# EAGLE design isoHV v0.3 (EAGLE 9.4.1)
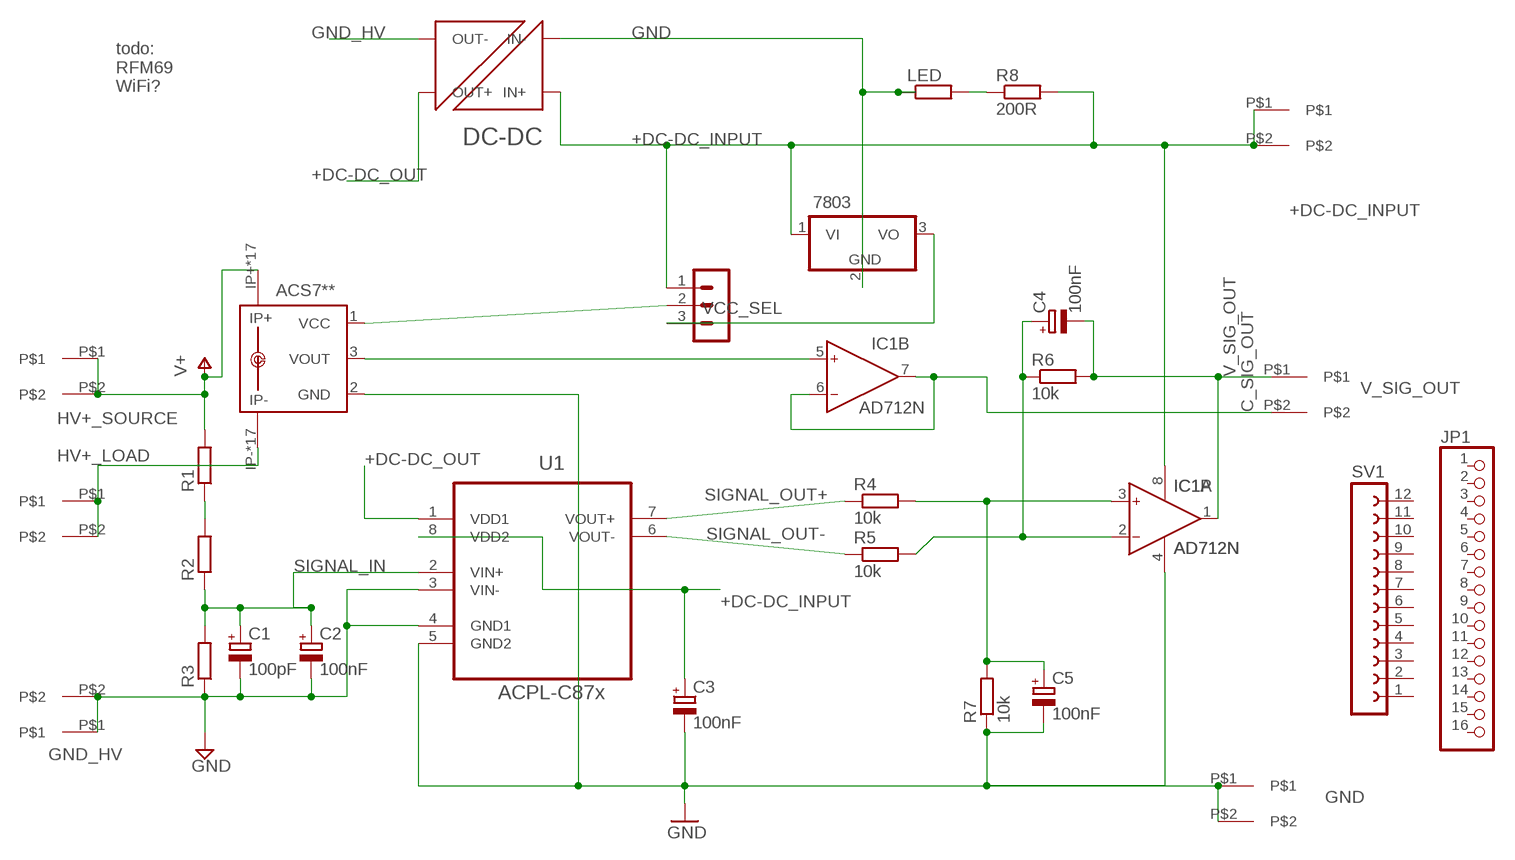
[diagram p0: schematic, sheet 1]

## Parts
7803  7805TV  [TO220V]
ACS7**  ACS758KCB-150B-PFF-T  [CB-PFF]
C1  100pF  CPOL-EUB45181A  [B45181A]
C2  100nF  CPOL-EUB45181A  [B45181A]
C3  100nF  CPOL-EUB45181A  [B45181A]
C4  100nF  CPOL-EUB45181A  [B45181A]
C5  100nF  CPOL-EUB45181A  [B45181A]
IC1  AD712N  [DIL08]
JP1  HEADER-1X16  [1X16_OVAL]
LED  R-EU_0204/2V  [0204V]
R1  R-EU_0411/15  [0411/15]
R2  R-EU_0411/15  [0411/15]
R3  R-EU_0411/15  [0411/15]
R4  10k  R-EU_0204/7  [0204/7]
R5  10k  R-EU_0204/7  [0204/7]
R6  10k  R-EU_0204/7  [0204/7]
R7  10k  R-EU_0204/7  [0204/7]
R8  200R  R-EU_0204/2V  [0204V]
SV1  FE12-1  [FE12]
U1  ACPL-C87x  ACPL-C79B-000E  [SOIC127P1150X330-8N]
U$1  7.62MM_TERMINAL_BLOCK  [7.62MM]
U$2  7.62MM_TERMINAL_BLOCK  [7.62MM]
U$3  7.62MM_TERMINAL_BLOCK  [7.62MM]
U$4  7.62MM_TERMINAL_BLOCK  [7.62MM]
U$5  7.62MM_TERMINAL_BLOCK  [7.62MM]
U$6  7.62MM_TERMINAL_BLOCK  [7.62MM]
U$7  NXF1  [NXF1]
VCC_SEL  MA03-1  [MA03-1]

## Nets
+DC-DC_INPUT: 7803.1(VI) C3.+ IC1.8(P:V+) R8.2 U1.8(VDD2) U$3.P$1 U$3.P$2 U$7.P$3(IN+) VCC_SEL.1
+DC-DC_OUT: U1.1(VDD1) U$7.P$8(OUT+)
C_SIG_OUT: IC1.6(B:IN-) IC1.7(B:OUT) U$5.P$2
GND: 7803.2(GND) ACS7**.2(GND) C3.- C5.- IC1.4(P:V-) LED.1 R7.1 U1.5(GND2) U$4.P$1 U$4.P$2 U$7.P$1(IN-)
GND_HV: C1.- C2.- R3.1 U1.3(VIN-) U1.4(GND1) U$2.P$1 U$2.P$2 U$7.P$7(OUT-) ; supply symbol labelled GND
HV+_LOAD: ACS7**.IP- ACS7**.IP-@2(IP-) ACS7**.IP-@3(IP-) ACS7**.IP-@4(IP-) ACS7**.IP-@5(IP-) ACS7**.IP-@6(IP-) ACS7**.IP-@7(IP-) ACS7**.IP-@8(IP-) ACS7**.IP-@9(IP-) ACS7**.IP-@10(IP-) ACS7**.IP-@11(IP-) ACS7**.IP-@12(IP-) ACS7**.IP-@13(IP-) ACS7**.IP-@14(IP-) ACS7**.IP-@15(IP-) ACS7**.IP-@16(IP-) ACS7**.IP-@17(IP-) U$6.P$1 U$6.P$2
HV+_SOURCE: ACS7**.IP+ ACS7**.IP+@2(IP+) ACS7**.IP+@3(IP+) ACS7**.IP+@4(IP+) ACS7**.IP+@5(IP+) ACS7**.IP+@6(IP+) ACS7**.IP+@7(IP+) ACS7**.IP+@8(IP+) ACS7**.IP+@9(IP+) ACS7**.IP+@10(IP+) ACS7**.IP+@11(IP+) ACS7**.IP+@12(IP+) ACS7**.IP+@13(IP+) ACS7**.IP+@14(IP+) ACS7**.IP+@15(IP+) ACS7**.IP+@16(IP+) ACS7**.IP+@17(IP+) R1.2 U$1.P$1 U$1.P$2 ; supply symbol labelled V+
N$1: C5.+ IC1.3(A:IN+) R4.2 R7.2
N$2: R1.1 R2.2
N$3: ACS7**.1(VCC) VCC_SEL.2
N$4: LED.2 R8.1
N$5: C4.+ IC1.2(A:IN-) R5.2 R6.1
N$6: ACS7**.3(VOUT) IC1.5(B:IN+)
N$7: 7803.3(VO) VCC_SEL.3
SIGNAL_IN: C1.+ C2.+ R2.1 R3.2 U1.2(VIN+)
SIGNAL_OUT+: R4.1 U1.7(VOUT+)
SIGNAL_OUT-: R5.1 U1.6(VOUT-)
V_SIG_OUT: C4.- IC1.1(A:OUT) R6.2 U$5.P$1
Unconnected: JP1.1 JP1.2 JP1.3 JP1.4 JP1.5 JP1.6 JP1.7 JP1.8 JP1.9 JP1.10 JP1.11 JP1.12 JP1.13 JP1.14 JP1.15 JP1.16 SV1.1 SV1.2 SV1.3 SV1.4 SV1.5 SV1.6 SV1.7 SV1.8 SV1.9 SV1.10 SV1.11 SV1.12

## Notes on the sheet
- todo:
  RFM69
  WiFi?

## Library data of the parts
7803 = linear:78*: Positive VOLTAGE REGULATOR Source: http://cache.national.com/ds/LM/LM78L05.pdf http://www.fairchildsemi.com/ds/LM/LM7805.pdf
ACS7** = allegro:ACS758*: Thermally Enhanced, Fully Integrated, Hall Effect-Based Linear Current Sensor with 100 micro Ohm Current Conductor display layer 49 Reference in BRD and place VIAs on circles Source: http://www.allegromicro.com/en/Products/Part_Numbers/0758/0758.pdf; MPN: ACS7**; OC_FARNELL: 1718995; OC_NEWARK: 04R7129
C1-C5 = rcl:CPOL-EU: POLARIZED CAPACITOR, European symbol; SPICEPREFIX: C
IC1 = analog-devices:AD712: Dual Precision, Low Cost, High Speed BiFET Op Amp Source: http://www.analog.com/static/imported-files/data_sheets/AD712.pdf; MF: ALTERA CORPORATION; MPN: AD712JNZ; OC_FARNELL: 9604898; OC_NEWARK: 59K4554
JP1 = microbuilder:HEADER-1X16: PIN HEADER
LED R1-R8 = rcl:R-EU_: RESISTOR, European symbol; SPICEPREFIX: R
SV1 = con-lsta-RFM69Pi:FE12-1: FEMALE HEADER; OC_FARNELL: unknown; OC_NEWARK: unknown
U1 = Avago_By_element14_Batch_1:ACPL-C79B-000E: Precision Miniature Isolation Amplifiers; DESCRIPTION: Precision Miniature Isolation Amplifiers; MPN: ACPL-C79B-000E; OC_FARNELL: 1854253; OC_NEWARK: 74R5803; PACKAGE: SOIC-8; SUPPLIER: AVAGO TECHNOLOGIES
U$1-U$6 = 7.62mm terminal block:7.62MM_TERMINAL_BLOCK
U$7 = NXF1:NXF1
VCC_SEL = con-lstb:MA03-1: PIN HEADER; OC_FARNELL: unknown; OC_NEWARK: unknown

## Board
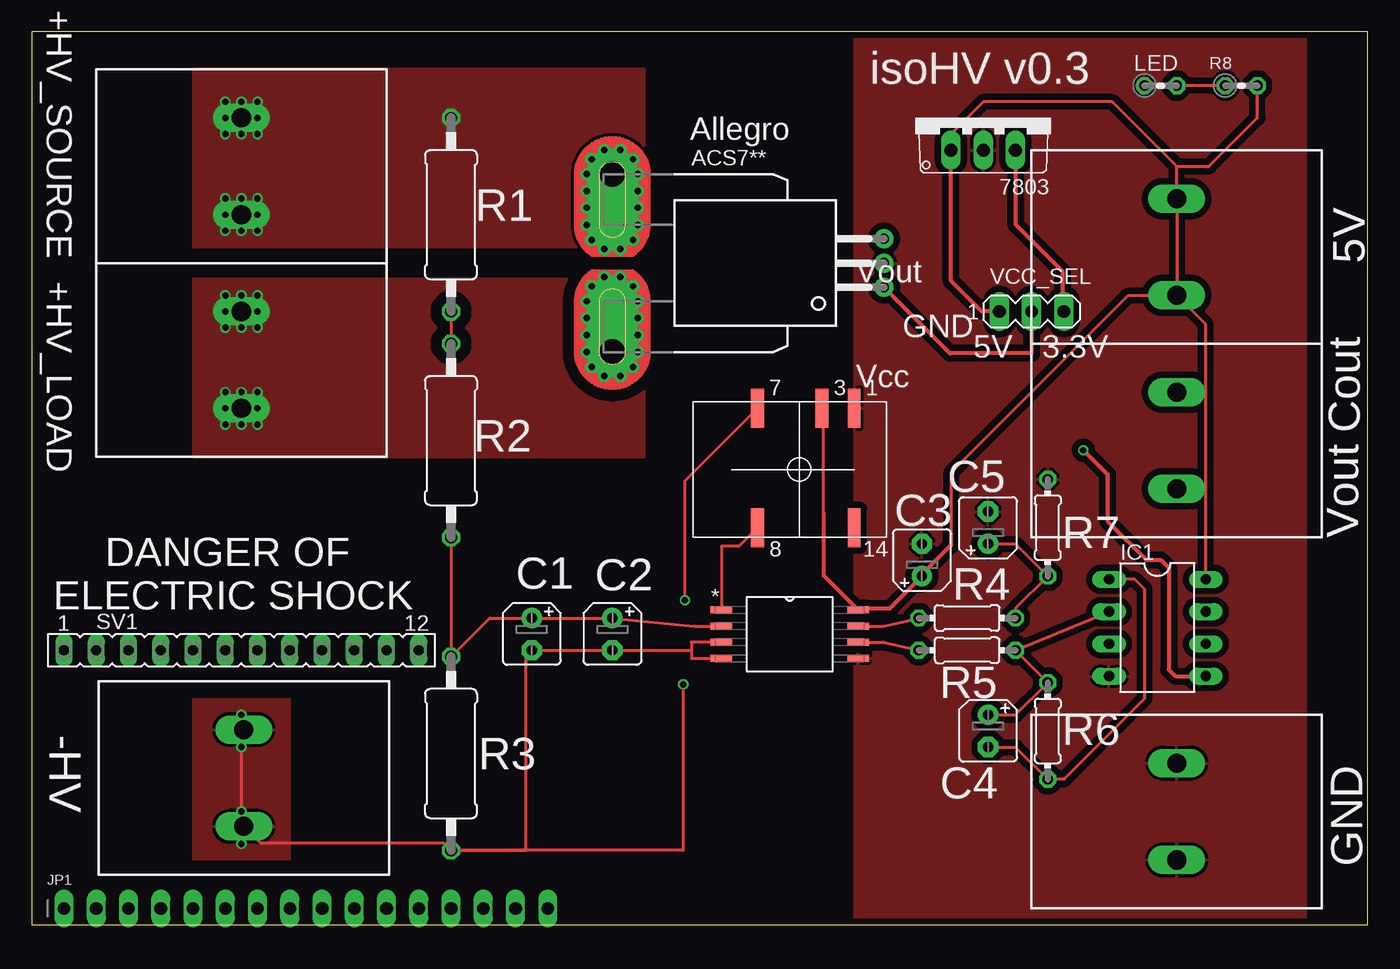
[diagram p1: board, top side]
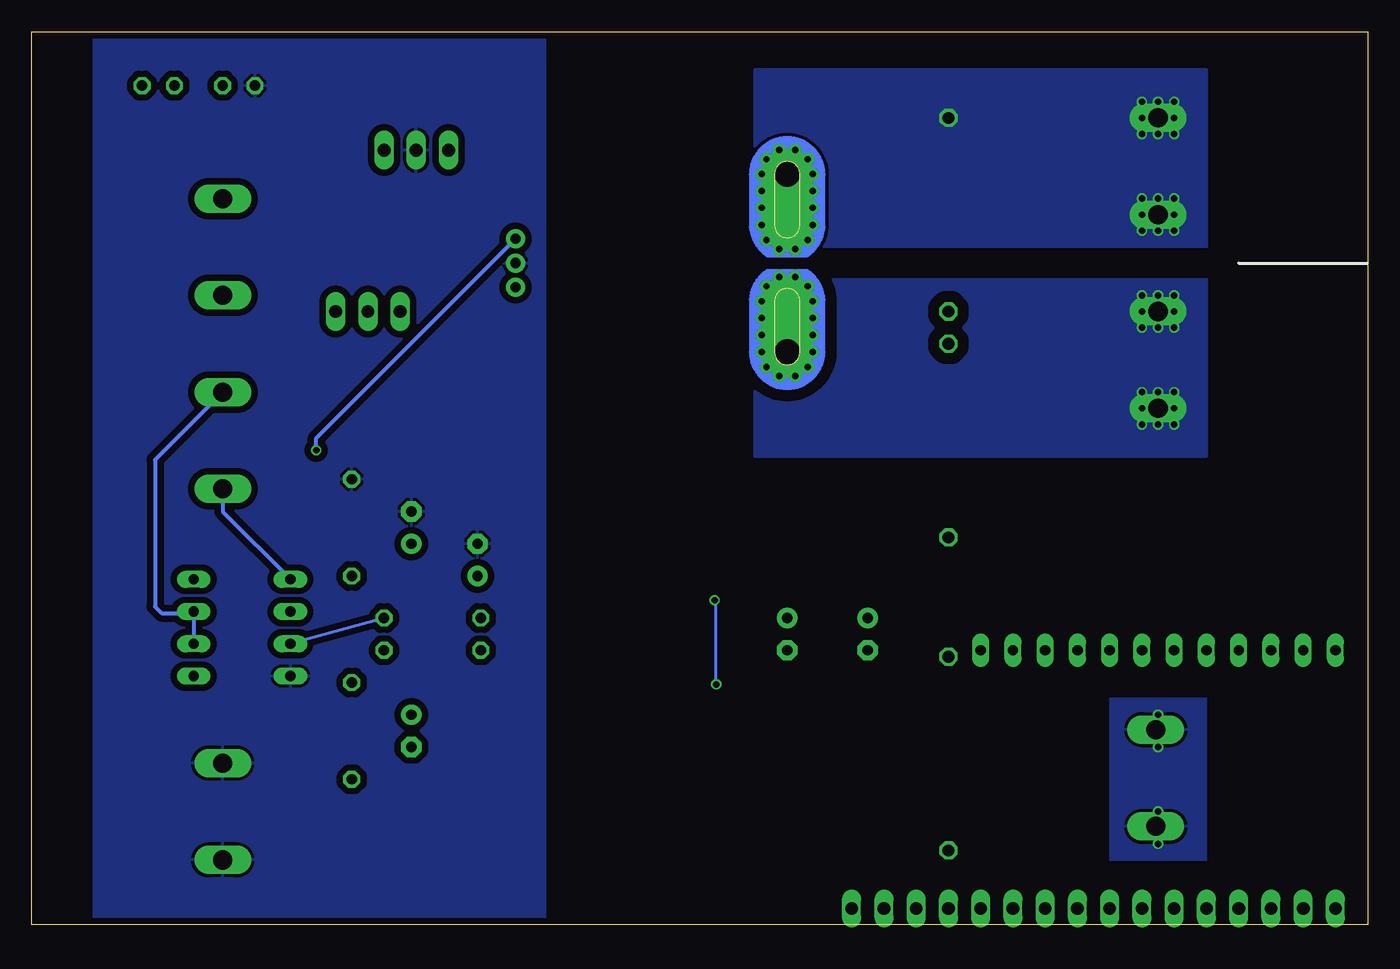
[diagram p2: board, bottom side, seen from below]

Size 105.21 x 70.28 mm. Coordinates in mm from the lower left corner, seen from the top.
Outline: 0,70.28 0,0 105.21,0 105.21,70.28 0,70.28
Copper layers (1*16): Top 0.07111875mm / dielectric 1.45776875mm / Bottom 0.07111875mm
Design rules "jlcpcb *": minimum track width 6mil, minimum drill 12mil, track to track 10mil, track to pad 10mil, pad to pad 10mil, via to via 10mil, smd to smd 0mil, copper to edge 10mil, drill to drill 10mil, minimum pad ring 10mil, minimum via ring 6mil, stop-mask expansion 2mil, vias tented up to drill 25mil, thermal gap 10mil

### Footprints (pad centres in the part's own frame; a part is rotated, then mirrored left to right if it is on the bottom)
TO220V = drill 1.016 long: 1 -2.54,-2.54; 2 0,-2.54; 3 2.54,-2.54
CB-PFF = drill 0.8 pad 1.5: 1 -1.91,-21.4; 2 0,-21.4; 3 1.91,-21.4 | drill 2 pad 4 offset: IP+ 7,0; IP- -7,0 | drill 0.5 pad 0.9: IP+@2 8.89,0.635; IP+@3 8.89,-0.635; IP+@4 8.175,-1.625; IP+@5 7,-2; IP+@6 5.675,-2; IP+@7 4.35,-2; IP+@8 3,-2; IP+@9 1.825,-1.625; IP+@10 1.1,-0.625; IP+@11 1.1,0.625; IP+@12 1.825,1.625; IP+@13 3,2; IP+@14 4.35,2; IP+@15 5.675,2; IP+@16 7,2; IP+@17 8.175,1.625; IP-@2 -8.89,0.635; IP-@3 -8.89,-0.635; IP-@4 -8.175,-1.625; IP-@5 -7,-2; IP-@6 -5.675,-2; IP-@7 -4.325,-2; IP-@8 -3,-2; IP-@9 -1.825,-1.625; IP-@10 -1.1,-0.625; IP-@11 -1.1,0.625; IP-@12 -1.825,1.625; IP-@13 -3,2; IP-@14 -4.325,2; IP-@15 -5.675,2; IP-@16 -7,2; IP-@17 -8.175,1.625
B45181A = drill 0.813 pad 1.6: + -1.27,0 | drill 0.813 pad 1.6 octagon: - 1.27,0
DIL08 = drill 0.813 long: 1 -3.81,-3.81; 2 -1.27,-3.81; 3 1.27,-3.81; 4 3.81,-3.81; 5 3.81,3.81; 6 1.27,3.81; 7 -1.27,3.81; 8 -3.81,3.81
1X16_OVAL = drill 1 long: 1 -19.05,0; 2 -16.51,0; 3 -13.97,0; 4 -11.43,0; 5 -8.89,0; 6 -6.35,0; 7 -3.81,0; 8 -1.27,0; 9 1.27,0; 10 3.81,0; 11 6.35,0; 12 8.89,0; 13 11.43,0; 14 13.97,0; 15 16.51,0; 16 19.05,0
0204V = drill 0.813 octagon: 1 -1.27,0; 2 1.27,0
0411/15 = drill 0.914 octagon: 1 -7.62,0; 2 7.62,0
0204/7 = drill 0.813 octagon: 1 -3.81,0; 2 3.81,0
FE12 = drill 0.813 long: 1 -13.97,0; 2 -11.43,0; 3 -8.89,0; 4 -6.35,0; 5 -3.81,0; 6 -1.27,0; 7 1.27,0; 8 3.81,0; 9 6.35,0; 10 8.89,0; 11 11.43,0; 12 13.97,0
SOIC127P1150X330-8N = smd 1.702 x 0.559: 1 -5.385,1.905; 2 -5.385,0.635; 3 -5.385,-0.635; 4 -5.385,-1.905; 5 5.385,-1.905; 6 5.385,-0.635; 7 5.385,0.635; 8 5.385,1.905
7.62MM = drill 1.5 long: P$1 0,-3.81; P$2 0,3.81
NXF1 = smd 0.991 x 3.048: P$1 0,0; P$3 2.54,0; P$7 7.62,0; P$8 7.62,9.398; P$14 0,9.398
MA03-1 = drill 1.016 long: 1 -2.54,0; 2 0,0; 3 2.54,0

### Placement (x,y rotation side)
7803  74.93,63.5 0 top
ACS7**  45.72,52.07 90 top
C1  39.37,22.86 270 top
C2  45.72,22.86 270 top
C3  70.1,28.7 90 top
C4  75.31,15.24 270 top
C5  75.31,31.24 90 top
IC1  88.65,23.37 270 top
JP1  21.59,1.27 0 top
LED  88.9,66.04 0 top
R1  33.02,55.88 90 top
R2  33.02,38.1 90 top
R3  33.02,13.46 90 top
R4  73.66,24.13 0 top
R5  73.66,21.59 0 top
R6  80.01,15.24 270 top
R7  80.01,31.24 270 top
R8  95.25,66.04 0 top
SV1  16.51,21.59 0 top
U1  59.69,22.86 0 top
U$1  16.51,59.69 180 top
U$2  16.7,11.54 0 top
U$3  90.17,53.34 0 top
U$4  90.17,8.89 180 top
U$5  90.17,38.1 0 top
U$6  16.51,44.45 0 top
U$7  64.77,40.64 180 top
VCC_SEL  78.74,48.26 0 top

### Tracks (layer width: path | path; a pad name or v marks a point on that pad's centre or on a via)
+DC-DC_INPUT
  Top 0.254: 65.08,24.88 U1.8 | IC1.8 92.46,47.24 U$3.P$1 | U$3.P$1 U$3.P$2 90.17,59.69 | 72.39,30.73 72.39,35.56 86.36,49.53 U$3.P$1 | 90.17,59.69 85.09,64.77 74.93,64.77 72.39,62.23 7803.1 | 62.36,30.48 62.36,40.51 U$7.P$3 | 90.17,59.69 92.71,59.69 96.52,63.5 R8.2
  Top 0.305: 7803.1 72.39,50.67 74.8,48.26 VCC_SEL.1 | 72.39,30.73 72.39,29.84 70.1,27.56 C3.+ 67.55,24.88 65.08,24.88 | U1.8 62.36,27.48 62.36,30.48 62.36,32.37
+DC-DC_OUT
  Top 0.254: U1.1 54.3,29.77 55.68,29.77 U$7.P$8
C_SIG_OUT
  Bottom 0.305: U$5.P$2 95.5,36.58 95.5,25.02 95,24.51 92.58,24.51 IC1.7 IC1.6
GND
  pour Bottom (isolate 0.508): 100.33,71.12 100.33,0 64.77,0 64.77,71.12
  pour Top (isolate 0.508): 64.77,71.12 64.77,0 100.33,0 100.33,71.12
GND_HV  (via drill 0.5)
  Top 0.254: U1.3 51.94,22.23 51.94,21.59 | 51.94,21.59 51.94,20.95 U1.4 | U$2.P$2 16.7,14.16 v16.51,13.97 v16.51,8.89 16.7,8.7 U$2.P$1 18.04,6.39 32.47,6.39 R3.1 | R3.1 38.9,5.84 38.9,21.12 C1.- C2.- 51.94,21.59 | R3.1 51.31,5.84 v51.31,18.9 | v51.44,25.53 51.44,34.92 U$7.P$7
  Bottom 0.254: v51.31,18.9 51.31,25.4 v51.44,25.53
  other vias: 16.51,16.51 16.51,6.35
  pour Top: 12.7,17.78 20.32,17.78 20.32,5.08 12.7,5.08
  pour Bottom: 12.7,17.78 20.32,17.78 20.32,5.08 12.7,5.08
HV+_LOAD  (via drill 0.5)
  other vias: 16.51,46.99 15.24,49.53 16.51,49.53 17.78,49.53 17.78,48.26 17.78,46.99 15.24,46.99 15.24,48.26 17.78,41.91 17.78,40.64 17.78,39.37 16.51,39.37 15.24,39.37 15.24,40.64 15.24,41.91 16.51,41.91
  pour Bottom (isolate 0.889, no thermals): 48.26,50.8 12.7,50.8 12.7,36.83 48.26,36.83
  pour Top (isolate 0.889, no thermals): 48.26,50.8 12.7,50.8 12.7,36.83 48.26,36.83
HV+_SOURCE  (via drill 0.5)
  other vias: 15.24,57.15 16.51,57.15 17.78,57.15 17.78,55.88 17.78,54.61 16.51,54.61 15.24,54.61 15.24,55.88 16.51,62.23 17.78,62.23 17.78,63.5 17.78,64.77 16.51,64.77 15.24,64.77 15.24,63.5 15.24,62.23
  pour Top (no thermals): 46.99,48.26 48.26,49.53 48.26,48.26
  pour Bottom (no thermals): 12.7,53.34 48.26,53.34 48.26,67.31 12.7,67.31
  pour Top (no thermals): 12.7,53.34 48.26,53.34 48.26,67.31 12.7,67.31
N$1
  Top 0.254: R4.2 77.47,24.89 R7.2 77.47,29.97 C5.+
  Bottom 0.254: R4.2 IC1.3
N$2
  Top 0.254: R1.1 R2.2
N$3
  Top 0.305: VCC_SEL.2 78.74,44.96 72.32,44.96 ACS7**.1
N$4
  Top 0.254: R8.1 LED.2
N$5
  Top 0.254: IC1.2 R5.2 R6.1 77.47,16.51 C4.+
N$6  (via drill 0.5)
  Top 0.305: v82.8,37.34 84.71,35.43 84.71,31.75 87.76,28.7 88.9,28.7 89.53,28.07 89.53,20.07 90.04,19.56 IC1.5
  Bottom 0.305: v82.8,37.34 82.8,38.3 ACS7**.3
N$7
  Top 0.305: 7803.3 77.47,55.12 81.15,51.44 81.15,48.39 VCC_SEL.3
SIGNAL_IN
  Top 0.254: R2.1 R3.2 36.07,24.13 C1.+ C2.+ 52.2,23.5 U1.2
SIGNAL_OUT+
  Top 0.254: U1.7 67.06,23.5 R4.1
SIGNAL_OUT-
  Top 0.254: U1.6 67.06,22.23 R5.1
V_SIG_OUT
  Top 0.254: C4.- 77.47,13.97 R6.2 81.28,11.43 87.63,17.78 87.63,26.42 86.87,27.18 IC1.1
  Bottom 0.305: U$5.P$1 90.17,32.51 IC1.1

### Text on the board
tNames: +HV_SOURCE | isoHV v0.3 | Allegro | 5V | +HV_LOAD | Vout | GND | 5V | 3.3V | Vcc | Cout | Vout | DANGER OF / ELECTRIC SHOCK | -HV | GND

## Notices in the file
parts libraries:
microbuilder: This work is placed in the public domain, and may be freely used for commercial and non-commercial work with the following conditions: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
